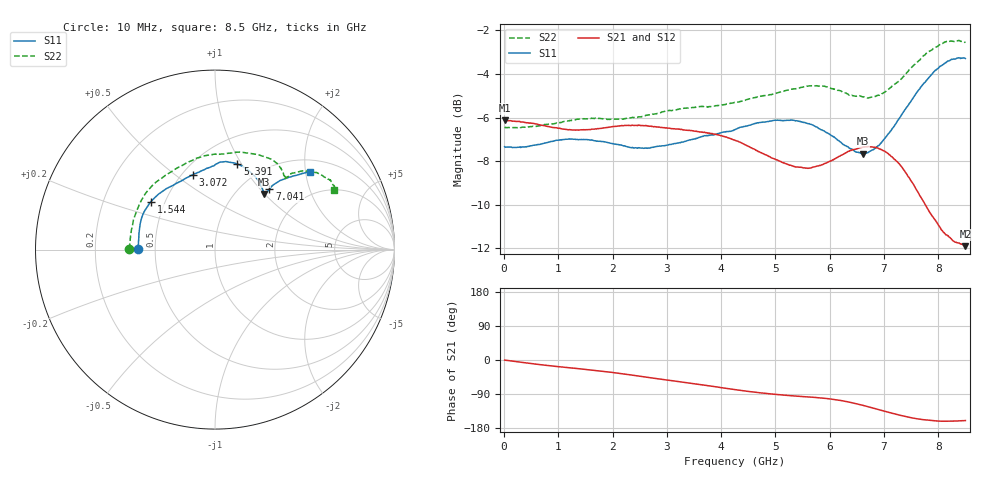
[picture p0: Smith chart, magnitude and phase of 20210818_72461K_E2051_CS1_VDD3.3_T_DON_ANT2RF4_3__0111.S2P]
!Agilent Technologies,E5071C,MY46417908,A.11.23
!Date: Wed Aug 18 14:34:38 2021
!Data & Calibration Information:
!Freq	S11:SOLT2(ON)	S21:SOLT2(ON)	S12:SOLT2(ON)	S22:SOLT2(ON)
!PortZ  Port1:50+j0  Port2:50+j0
!Above PortZ is port z conversion or system Z0 setting when saving the data.
!When reading, reference impedance value at option line is always used.
# Hz S dB R 50
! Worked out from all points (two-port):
!   1601 points, 10 MHz to 8.5 GHz, reference 50 ohm
!   highest |S21| = -6.12 dB at 10 MHz (marker M1); lowest = -11.9 dB at 8.5 GHz (marker M2)
!   |S21| within 3 dB of the highest: start of sweep to 7.556 GHz
!   lowest |S11| = -7.7 dB at 6.606 GHz (marker M3), VSWR 2.41, Z = 66.5 + j49.8 ohm
!   |S11| at or under -10 dB: nowhere
!   |S22| runs from -6.5 to -2.5 dB; largest |S21 - S12| = 0.0015
!   S11 on the Smith chart (normalised r, x): 10 MHz: 0.40, +0.00; 1.544 GHz: 0.42, +0.28; 3.072 GHz: 0.57, +0.58; 5.391 GHz: 0.76, +0.96; 7.041 GHz: 1.33, +1.12; 8.5 GHz: 1.30, +2.13
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1e7  -7.33 179.6  -6.12 -0.4  -6.12 -0.3  -6.43 179.6
7.847125e8  -7.15 162.2  -6.40 -14.3  -6.39 -14.3  -6.31 159.2
1.426769e9  -7.00 146.3  -6.56 -23.7  -6.56 -23.6  -6.05 140.0
1.543506e9  -7.01 143.3  -6.56 -25.4  -6.56 -25.4  -6.05 136.6
2.185562e9  -7.29 127.2  -6.37 -36.5  -6.37 -36.5  -6.07 119.0
2.843538e9  -7.32 111.2  -6.43 -49.7  -6.43 -49.8  -5.80 104.3
3.071706e9  -7.23 106.4  -6.50 -54.2  -6.49 -54.2  -5.68 100.2
3.591719e9  -6.91 97.0  -6.65 -64.5  -6.64 -64.5  -5.49 90.9
4.255e9  -6.55 90.2  -7.04 -78.1  -7.03 -78.1  -5.31 81.8
4.790931e9  -6.21 85.7  -7.68 -87.7  -7.68 -87.6  -4.99 74.4
5.390538e9  -6.14 75.4  -8.26 -95.3  -8.27 -95.3  -4.66 62.7
5.671769e9  -6.33 68.6  -8.30 -98.1  -8.31 -98.1  -4.54 57.6
6.149331e9  -7.04 55.8  -7.82 -105.7  -7.83 -105.8  -4.75 49.8
6.435869e9  -7.50 50.5  -7.47 -113.6  -7.48 -113.7  -5.00 46.2
6.605669e9  -7.66 48.6  -7.36 -119.4  -7.36 -119.5  -5.04 45.9
6.839144e9  -7.41 48.1  -7.38 -128.4  -7.39 -128.4  -5.03 45.3
7.040781e9  -6.87 48.0  -7.59 -136.4  -7.60 -136.4  -4.78 45.0
7.088538e9  -6.72 48.1  -7.68 -138.3  -7.70 -138.3  -4.68 44.9
7.380381e9  -5.65 46.9  -8.45 -148.7  -8.45 -148.8  -4.05 43.4
7.788962e9  -4.28 42.5  -10.12 -158.6  -10.11 -158.7  -3.04 37.5
8.123256e9  -3.50 40.0  -11.33 -161.5  -11.30 -161.5  -2.53 31.5
8.5e9  -3.29 39.2  -11.90 -159.7  -11.89 -159.9  -2.57 26.7
